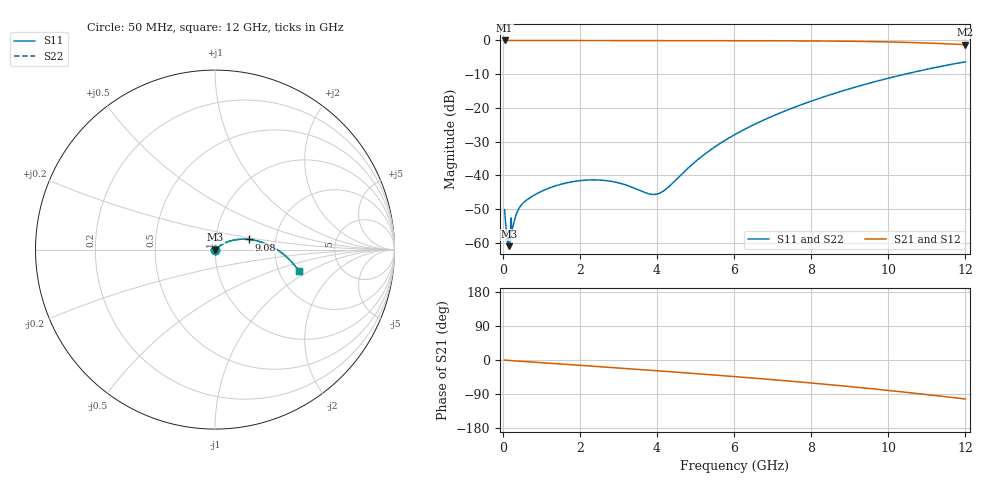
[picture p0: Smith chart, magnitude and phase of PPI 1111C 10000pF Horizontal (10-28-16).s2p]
# MHz S MA R 50
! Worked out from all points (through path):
!   1601 points, 50 MHz to 12 GHz, reference 50 ohm
!   highest |S21| = 0.00 dB at 50 MHz (marker M1); lowest = -1.3 dB at 12 GHz (marker M2)
!   group delay of S21, straight-line fit = 23.3 ps
!   lowest |S11| = -61.1 dB at 169.5 MHz (marker M3), VSWR 1.00, Z = 50.1 - j0.0346 ohm
!   |S11| at or under -10 dB: start of sweep to 10.44 GHz
!   |S22| runs from -61.1 to -6.3 dB; largest |S21 - S12| = 0
!   S11 on the Smith chart (normalised r, x): 50 MHz: 1.00, -0.01; 9.08 GHz: 1.46, +0.17; 12 GHz: 2.57, -0.80
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50  0.003079 -83.4  0.9996 -0.2  0.9996 -0.2  0.003079 -83.4
132.1562  0.001089 -36.6  0.9991 -0.9  0.9991 -0.9  0.001089 -36.6
147.0938  0.0009823 -45.4  0.9993 -1.0  0.9993 -1.0  0.0009823 -45.4
169.5  0.000885 -23.0  0.9992 -1.2  0.9992 -1.2  0.000885 -23.0
214.3125  0.002235 8.3  0.9978 -1.6  0.9978 -1.6  0.002235 8.3
266.5938  0.00171 -5.6  0.9983 -1.9  0.9983 -1.9  0.00171 -5.6
393.5625  0.002996 -13.0  0.997 -2.8  0.997 -2.8  0.002996 -13.0
617.625  0.004264 -35.0  0.9963 -4.3  0.9963 -4.3  0.004264 -35.0
1267.406  0.006643 -61.4  0.9959 -8.9  0.9959 -8.9  0.006643 -61.4
2044.156  0.008356 -72.9  0.9955 -14.3  0.9955 -14.3  0.008356 -72.9
2820.906  0.008102 -74.5  0.9951 -19.8  0.9951 -19.8  0.008102 -74.5
3784.375  0.005306 -42.4  0.9947 -26.8  0.9947 -26.8  0.005306 -42.4
4038.312  0.005324 -18.1  0.9945 -28.6  0.9945 -28.6  0.005324 -18.1
4269.844  0.006449 3.6  0.9944 -30.4  0.9944 -30.4  0.006449 3.6
5203.438  0.01979 35.4  0.9937 -37.4  0.9937 -37.4  0.01979 35.4
6025  0.04018 37.0  0.9925 -43.8  0.9925 -43.8  0.04018 37.0
6936.188  0.07263 33.1  0.99 -51.3  0.99 -51.3  0.07263 33.1
8019.156  0.1267 25.6  0.9836 -60.8  0.9836 -60.8  0.1267 25.6
9079.719  0.198 16.5  0.9708 -70.9  0.9708 -70.9  0.198 16.5
10013.31  0.2763 7.5  0.9507 -80.4  0.9507 -80.4  0.2763 7.5
10999.19  0.3733 -2.9  0.9162 -91.2  0.9162 -91.2  0.3733 -2.9
12000  0.4816 -14.3  0.8638 -102.8  0.8638 -102.8  0.4816 -14.3
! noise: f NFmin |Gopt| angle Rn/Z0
50  0.0004129  0.8785  0.3639  0.0007347
1372  0.007241  0.8173  9.922  0.008232
2701  0.01075  0.7687  19.38  0.009201
4031  0.01378  0.7428  28.54  0.01011
5360  0.01664  0.7302  37.27  0.01106
6682  0.01947  0.727  45.46  0.01212
8012  0.0224  0.7307  53.15  0.01334
9341  0.02552  0.7398  60.27  0.01481
1.067e+04  0.02893  0.753  66.86  0.0166
1.2e+04  0.03272  0.7691  72.94  0.01884
